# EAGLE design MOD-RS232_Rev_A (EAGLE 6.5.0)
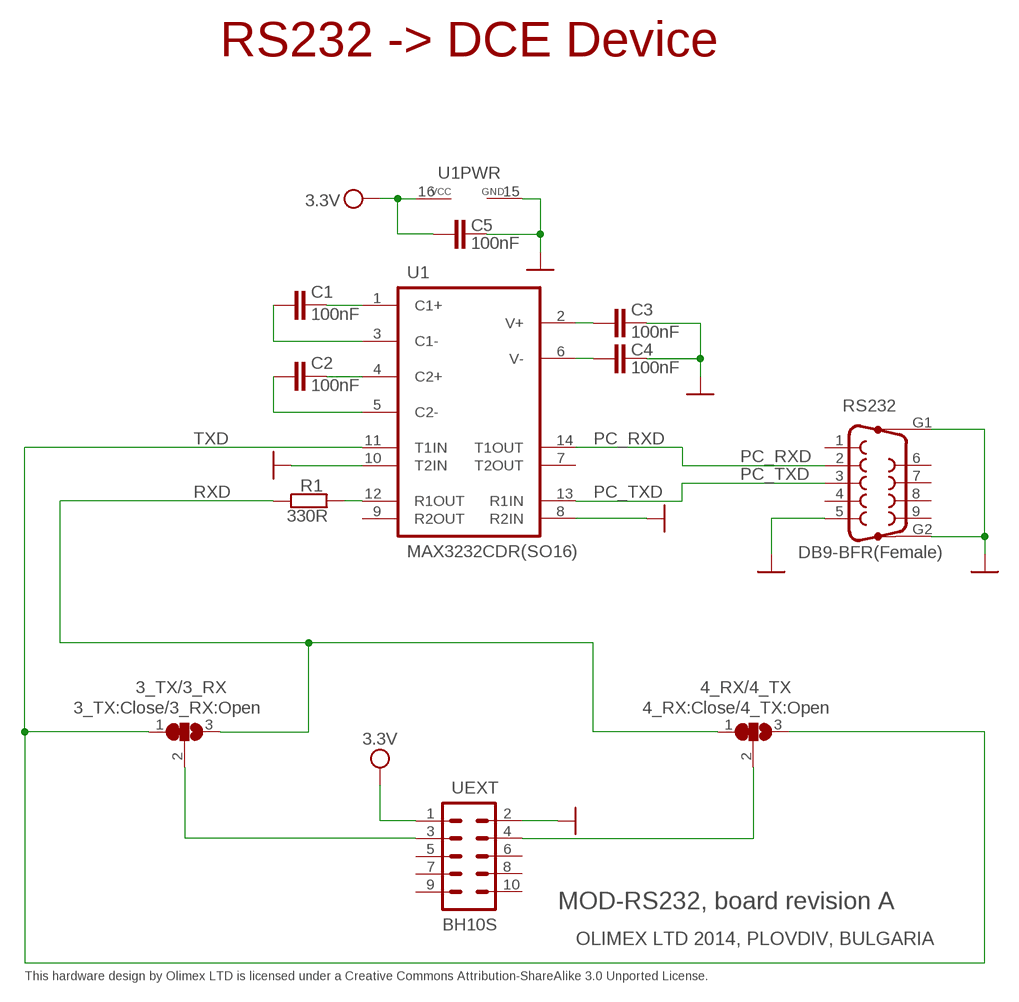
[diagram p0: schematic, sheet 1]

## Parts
3_TX/3_RX  3_TX:Close/3_RX:Open  SJ2W3  [SJ_2_SMALL]
4_RX/4_TX  4_RX:Close/4_TX:Open  SJ2W3  [SJ_2_SMALL]
C1  100nF  C-EUC0603_DWS  [C0603_DWS]
C2  100nF  C-EUC0603_DWS  [C0603_DWS]
C3  100nF  C-EUC0603_DWS  [C0603_DWS]
C4  100nF  C-EUC0603_DWS  [C0603_DWS]
C5  100nF  C-EUC0603_DWS  [C0603_DWS]
R1  330R  R-EU_R0603_5MIL_DWS  [R0603_5MIL_DWS]
RS232  DB9-BFR(Female)  F09HP_DB9-BFR  [DB9-BFR]
U1  MAX3232CDR(SO16)  MAX32321  [SO16-150MIL-THIN_PADS]
UEXT  BH10S  ML10  [ML10-MALE]

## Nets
GND: C3.2 C4.2 C5.2 RS232.5 RS232.G1 RS232.G2 U1.8(R2IN) U1.10(T2IN) U1.15(GND) UEXT.2
N$1: 3_TX/3_RX.2 UEXT.3
N$2: 4_RX/4_TX.2 UEXT.4
N$31: C1.1 U1.3(C1-)
N$44: C2.1 U1.5(C2-)
N$45: C1.2 U1.1(C1+)
N$46: C2.2 U1.4(C2+)
N$47: C4.1 U1.6(V-)
N$48: C3.1 U1.2(V+)
N$69: R1.2 U1.12(R1OUT)
PC_RXD: RS232.2 U1.14(T1OUT)
PC_TXD: RS232.3 U1.13(R1IN)
RXD: 3_TX/3_RX.3 4_RX/4_TX.1 R1.1
TXD: 3_TX/3_RX.1 4_RX/4_TX.3 U1.11(T1IN)
VCC: C5.1 U1.16(VCC) UEXT.1 ; supply symbol labelled 3.3V
Unconnected: RS232.1 RS232.4 RS232.6 RS232.7 RS232.8 RS232.9 U1.7(T2OUT) U1.9(R2OUT) UEXT.5 UEXT.6 UEXT.7 UEXT.8 UEXT.9 UEXT.10

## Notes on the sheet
- RS232 -> DCE Device
- MOD-RS232, board revision A
- OLIMEX LTD 2014, PLOVDIV, BULGARIA
- This hardware design by Olimex LTD is licensed under a Creative Commons Attribution-ShareAlike 3.0 Unported License.

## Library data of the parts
3_TX/3_RX 4_RX/4_TX = jumper:SJ2W: SMD solder JUMPER
C1-C5 = rcl:C-EU: CAPACITOR, European symbol
R1 = rcl:R-EU_: RESISTOR, European symbol
RS232 = con-subd:F09HP: SUB-D
U1 = gogo:MAX3232
UEXT = con-harting-ml:ML10: HARTING

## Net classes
1 pwr: width 0.254 mm
2 thin: width 0.025 mm, clearance 0.025 mm

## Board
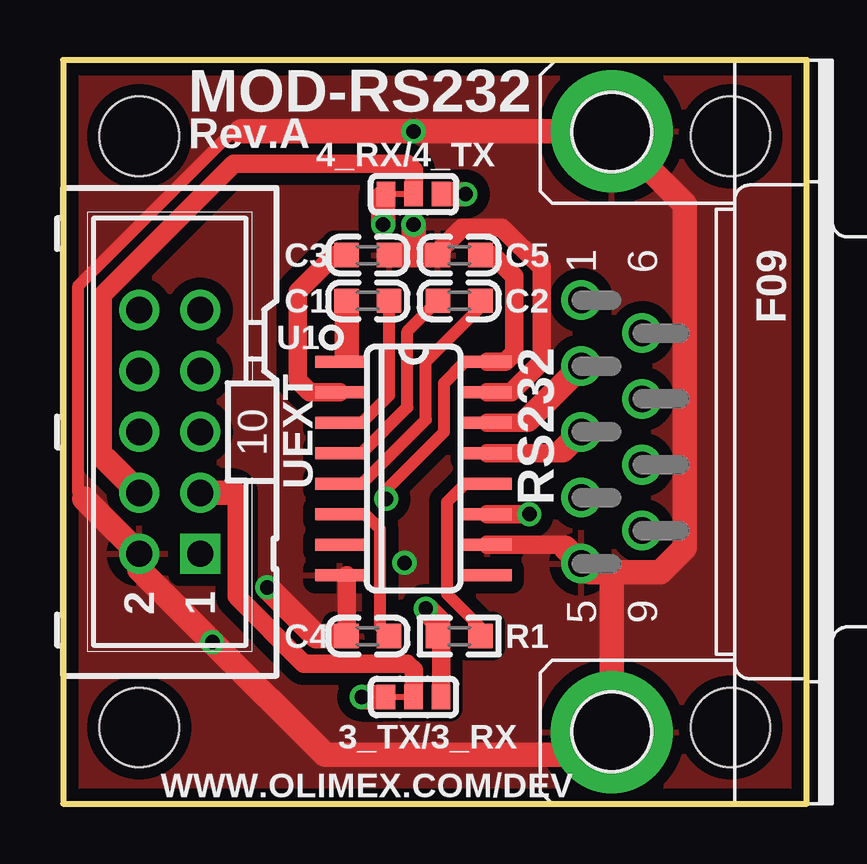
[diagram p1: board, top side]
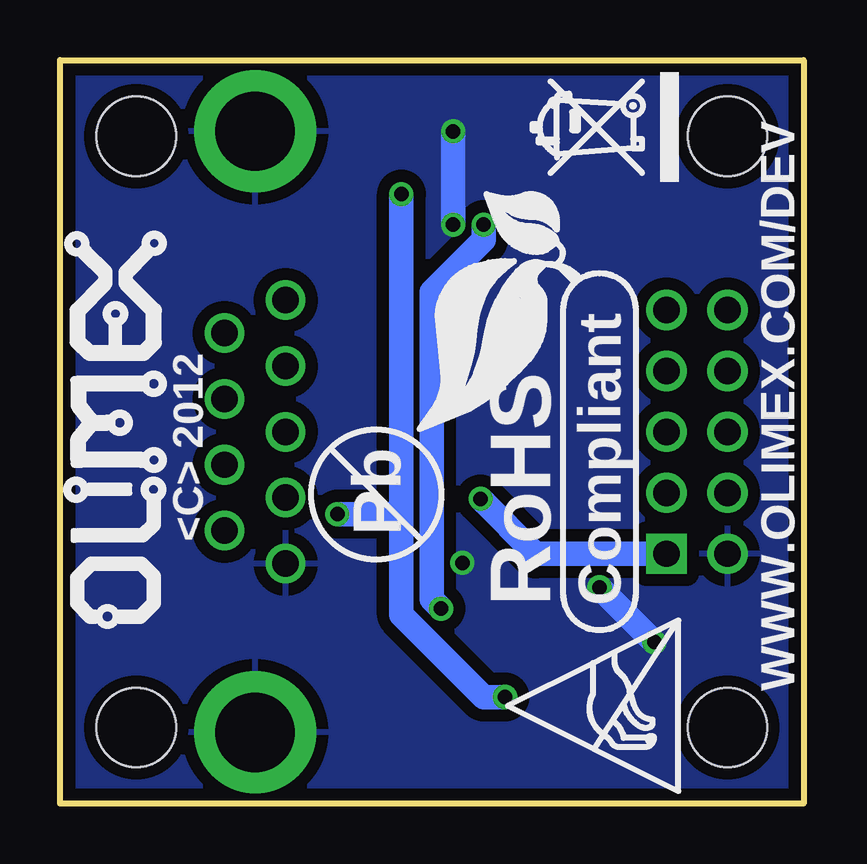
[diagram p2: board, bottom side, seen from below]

Size 30.99 x 30.99 mm. Coordinates in mm from the lower left corner, seen from the top.
Outline: 0,0 30.99,0 30.99,30.99 0,30.99 0,0
Copper layers (1+16): Top 0.035mm / dielectric 1.5mm / Bottom 0.035mm
Design rules "default": minimum track width 10mil, minimum drill 23mil, track to track 9.5mil, track to pad 9.5mil, pad to pad 9.5mil, via to via 10mil, smd to smd 0mil, copper to edge 8mil, drill to drill 8mil, minimum pad ring 10mil, minimum via ring 8mil, stop-mask expansion 4mil, vias tented up to drill 25mil, thermal gap 20mil
Holes 3.3 mm at 3.17,27.81 3.17,3.17 27.81,3.17 27.81,27.81

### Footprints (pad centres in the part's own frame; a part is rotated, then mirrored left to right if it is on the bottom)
SJ_2_SMALL = smd 0.762 x 1.016: 1 -1.143,0; 2 0,0; 3 1.143,0
C0603_DWS = smd 1.016 x 1.016: 1 -0.889,0; 2 0.889,0
R0603_5MIL_DWS = smd 1.016 x 1.016: 1 -0.889,0; 2 0.889,0
DB9-BFR = drill 1.1: 1 -5.486,-1.27; 2 -2.743,-1.27; 3 0,-1.27; 4 2.743,-1.27; 5 5.486,-1.27; 6 -4.115,1.27; 7 -1.372,1.27; 8 1.372,1.27; 9 4.115,1.27 | drill 3.302 pad 5.08: G1 -12.522,0; G2 12.522,0
SO16-150MIL-THIN_PADS = smd 0.508 x 2.032: 1 -4.445,-3.073; 2 -3.175,-3.073; 3 -1.905,-3.073; 4 -0.635,-3.073; 5 0.635,-3.073; 6 1.905,-3.073; 7 3.175,-3.073; 8 4.445,-3.073; 9 4.445,3.073; 10 3.175,3.073; 11 1.905,3.073; 12 0.635,3.073; 13 -0.635,3.073; 14 -1.905,3.073; 15 -3.175,3.073; 16 -4.445,3.073
ML10-MALE = drill 1.1 pad 1.676 square: 1 -5.08,-1.27 | drill 1.1 pad 1.676: 2 -5.08,1.27; 3 -2.54,-1.27; 4 -2.54,1.27; 5 0,-1.27; 6 0,1.27; 7 2.54,-1.27; 8 2.54,1.27; 9 5.08,-1.27; 10 5.08,1.27

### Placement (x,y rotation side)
3_TX/3_RX  14.61,4.45 0 top
4_RX/4_TX  14.61,25.4 0 top
C1  12.7,20.95 180 top
C2  16.51,20.95 180 top
C3  12.7,22.86 0 top
C4  12.7,6.99 180 top
C5  16.51,22.86 180 top
R1  16.51,6.99 0 top
RS232  22.86,15.49 270 top
U1  14.61,13.97 270 top
U$1  [OLIMEX_LOGO1_V]  26.42,25.02 90 bottom
U$8  [RECYCLE_BIN1/8]  5.21,25.91 90 bottom
U$9  [PB]  17.81,12.88 90 bottom
U$10  [ESD_SYMBOL]  5.22,0.52 90 bottom
U$13  [ROHS]  7.62,8.26 90 bottom
UEXT  4.45,15.49 90 top

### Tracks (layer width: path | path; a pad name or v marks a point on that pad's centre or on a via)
GND  (via drill 0.6)
  Top 0.508: 11.81,9.53 U1.8 | 7.42,28.02 7.06,28.02 0.64,21.59 0.64,12.95 0.89,12.7
  Top 0.762: 20.93,10.67 20.8,10.79 U1.10 | C4.2 11.81,9.53 | U1.15 18.67,17.14 19.94,18.41 19.94,22.35 18.29,24 16.64,24 15.62,22.99 C5.2
  Top 1.016: 20.93,10.67 RS232.5 21.95,9.65 22.86,9.65 | 22.86,9.65 24.89,9.65 25.91,10.67 25.91,24.97 RS232.G1 v14.61,28.02 7.42,28.02 | 22.86,9.65 RS232.G2 21.92,2.03 10.92,2.03 v6.22,6.73 3.17,9.78 UEXT.2 0.89,12.7 | 14.61,22.86 C5.2 | v14.61,24.13 14.61,22.86 | 14.61,22.86 C3.2 | v8.51,9.02 10.54,6.99 C4.2
  Bottom 1.016: v14.61,28.02 v14.61,24.13 | v6.22,6.73 v8.51,9.02
  other vias: 14.22,10.03
  pour Top (isolate 0.508): -2.54,-2.54 34.29,-2.54 34.29,2.54 34.29,34.29 27.94,34.29 -2.54,34.29
  pour Bottom (isolate 0.508): -5.08,-5.08 36.83,-5.08 36.83,-1.27 36.83,36.83 33.02,36.83 -5.08,36.83
N$1
  Top 0.254: 3_TX/3_RX.2 13.59,4.45
  Top 0.762: 3_TX/3_RX.2 14.61,5.59 14.35,5.84 10.03,5.84 7.24,8.64 7.24,12.95 7.11,12.95
  Top 1.016: 7.11,12.95 UEXT.3
N$2
  Top 0.254: 4_RX/4_TX.2 13.59,25.4
  Top 0.762: 1.78,14.35 1.65,14.48 1.65,21.21 7.11,26.67 14.35,26.67 14.61,26.42 4_RX/4_TX.2
  Top 1.016: 1.78,14.35 UEXT.4
N$31
  Top 0.508: U1.3 12.45,15.88 13.59,17.02 C1.1
N$44
  Top 0.508: U1.5 12.45,13.34 15.11,16 15.11,18.41 17.4,20.7 C2.1
N$45
  Top 0.508: U1.1 11.81,18.41 11.81,18.67
  Top 1.016: 11.81,18.67 C1.2
N$46
  Top 0.508: U1.4 12.45,14.61 14.35,16.51 14.35,19.68 C2.2
N$47
  Top 0.508: U1.6 12.57,12.06 13.21,11.43 13.21,7.37 C4.1
N$48
  Top 0.762: U1.2 10.29,17.14 9.78,17.65 9.78,21.34 11.3,22.86 C3.1
N$69
  Top 0.508: U1.12 16.76,13.34 16,12.57 16,8.74 17.4,7.34 R1.2
PC_RXD
  Top 0.762: U1.14 19.23,15.88 19.36,16
  Top 1.016: 19.36,16 RS232.2
PC_TXD
  Top 0.762: U1.13 20.7,14.61 20.83,14.73
  Top 1.016: 20.83,14.73 RS232.3
RXD  (via drill 0.6)
  Top 0.508: 13.34,25.27 4_RX/4_TX.1
  Top 0.762: 3_TX/3_RX.3 15.75,6.86 R1.1
  Top 1.016: R1.1 15.62,7.62 v15.11,8.13 | v13.34,24.13 13.34,25.27
  Bottom 1.016: v15.11,8.13 15.49,8.51 15.49,21.34 13.34,23.5 v13.34,24.13
TXD  (via drill 0.6)
  Top 0.508: 13.34,4.45 3_TX/3_RX.1 | 15.88,25.4 4_RX/4_TX.3
  Top 0.762: v19.43,12.06 U1.11
  Top 1.016: v12.45,4.45 13.34,4.45 | v16.76,25.4 15.88,25.4
  Bottom 1.016: v12.45,4.45 13.34,4.45 16.76,7.87 16.76,12.06 | 16.76,12.06 v19.43,12.06 | 16.76,12.06 v16.76,25.4
VCC  (via drill 0.6)
  Top 0.508: U1.16 16.76,18.41 15.88,17.53 15.88,15.49 13.46,13.08 v13.46,12.7
  Top 0.762: U1.16 18.41,18.41 18.8,18.8 18.8,21.97 17.91,22.86 C5.1
  Bottom 1.016: v13.46,12.7 11.18,10.41 UEXT.1

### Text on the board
tNames: MOD-RS232 | Rev.A | WWW.OLIMEX.COM/DEV
bNames: <C> 2012 | WWW.OLIMEX.COM/DEV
